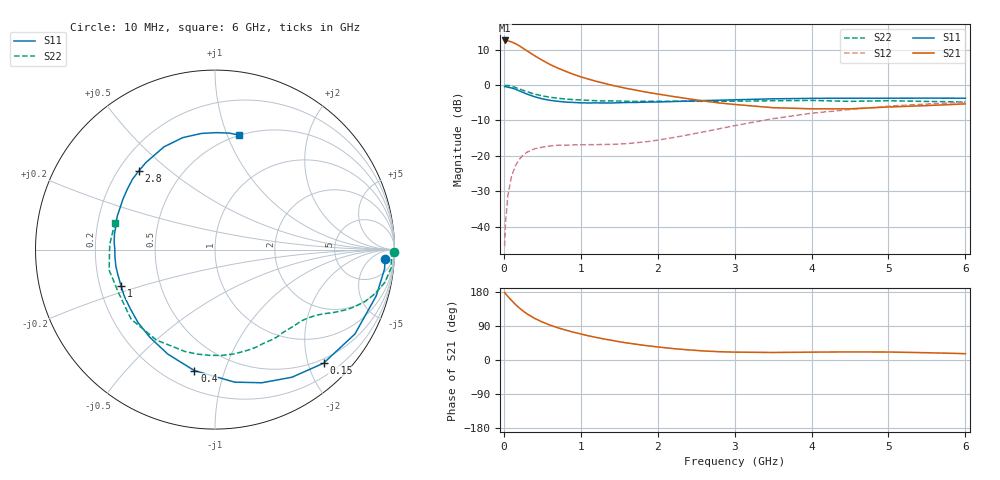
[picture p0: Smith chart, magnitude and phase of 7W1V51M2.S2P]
! Infineon Technologies  Discrete & RF Semiconductors
! BFS17W
! Si NPN RF Bipolar Junction Transistor in SOT323
! VCE = 1.5 V  IC = 1.2 mA
! Common Emitter S-Parameters:  August  1999
# GHz  S  MA  R  50
!  f  S11  S21  S12  S22
! GHz  MAG  ANG  MAG  ANG  MAG  ANG  MAG  ANG
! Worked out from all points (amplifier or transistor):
!   36 points, 10 MHz to 6 GHz, reference 50 ohm
!   highest |S21| = 12.6 dB at 10 MHz (marker M1)
!   |S21| within 3 dB of that: start of sweep to 306.7 MHz
!   unconditionally stable (mu >= 1): 933.2 MHz to end of sweep
!   at 250 MHz: K = 0.30, MSG = 15.1 dB, |S12| = -19.8 dB
!   at 1.4 GHz: K = 1.35, MAG = 4.8 dB, |S12| = -16.8 dB
!   at 6 GHz: K = 1.12, MAG = -2.4 dB, |S12| = -4.8 dB
!   S11 on the Smith chart (normalised r, x): 10 MHz: 18, -19; 150 MHz: 0.42, -2.27; 400 MHz: 0.31, -0.79; 1 GHz: 0.29, -0.17; 2.8 GHz: 0.28, +0.40; 6 GHz: 0.50, +1.11
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0.01  0.9481 -3.1  4.267 178.4  0.0053 85.7  0.9992 -0.7
0.02  0.951 -6.5  4.266 175.5  0.0104 93.6  0.9834 -2.2
0.05  0.9346 -16.0  4.226 168.2  0.0266 82.0  0.9874 -5.7
0.1  0.9104 -31.1  4.071 157.4  0.0515 71.8  0.9632 -11.0
0.15  0.8754 -46.3  3.847 146.7  0.0721 64.0  0.9234 -15.5
0.2  0.8304 -58.9  3.593 137.5  0.089 57.5  0.884 -19.1
0.25  0.7865 -70.6  3.305 129.3  0.1019 51.2  0.8425 -22.1
0.3  0.7465 -81.6  3.054 122.0  0.1124 46.9  0.8069 -24.5
0.4  0.6837 -99.7  2.597 109.8  0.1258 39.8  0.7454 -28.1
0.5  0.6388 -114.3  2.239 100.3  0.1328 35.0  0.7041 -30.5
0.6  0.609 -126.5  1.955 92.1  0.138 32.0  0.6731 -32.9
0.8  0.5756 -145.1  1.568 79.1  0.1419 29.3  0.635 -37.6
1  0.5611 -158.7  1.307 68.7  0.1436 28.9  0.6163 -42.2
1.1  0.5589 -165.4  1.214 63.8  0.1439 29.5  0.6083 -45.2
1.6  0.567 171.1  0.894 45.0  0.1487 37.1  0.5905 -60.0
2.2  0.585 151.2  0.69 30.1  0.1812 49.6  0.5909 -79.4
2.8  0.6105 133.8  0.559 21.9  0.2416 55.2  0.5905 -99.8
3.5  0.6392 116.4  0.479 19.8  0.3353 53.1  0.6006 -122.9
4  0.6492 106.1  0.462 20.7  0.4005 47.8  0.6072 -140.4
4.5  0.6516 96.7  0.462 21.4  0.4508 41.7  0.5889 -156.1
5.5  0.654 83.0  0.513 19.2  0.5398 29.9  0.5872 177.2
6  0.652 78.0  0.542 16.7  0.5743 24.3  0.5772 165.4
